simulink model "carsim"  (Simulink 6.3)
settings: Solver=ode3  StartTime=0.0  StopTime=130  RelTol=1e-3
libraries: simulink x2

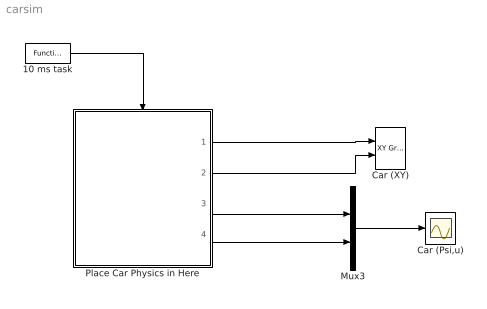
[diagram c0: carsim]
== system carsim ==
  10 ms task : simulink/Ports & Subsystems/Function-Call Generator  sample_time=0.01  numberOfIterations=1
  Car (Psi,u) : Scope
  Car (XY) : simulink/Sinks/XY Graph  xmin=-250  xmax=250  ymin=-250  ymax=250  st=-1
  Mux3 : Mux  Inputs=2
  Place Car Physics in Here : Subsystem  TreatAsAtomicUnit=on
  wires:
  10 ms task/1 -> Place Car Physics in Here/Trigger
  Place Car Physics in Here/3(psi) -> Mux3/1
  Place Car Physics in Here/1(x) -> Car (XY)/1
  Place Car Physics in Here/2(y) -> Car (XY)/2
  Place Car Physics in Here/4(u) -> Mux3/2
  Mux3/1 -> Car (Psi,u)/1

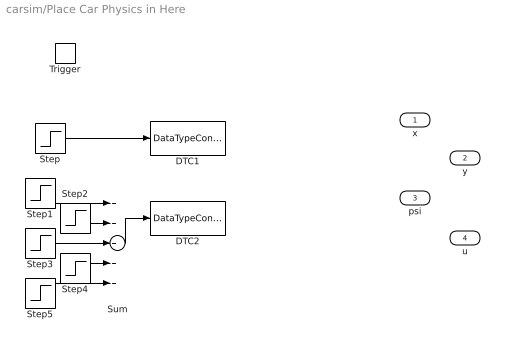
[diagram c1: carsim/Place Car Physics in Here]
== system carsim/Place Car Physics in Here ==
  Trigger : TriggerPort  TriggerType=function-call
  DTC1 : DataTypeConversion  OutDataTypeMode=single
  DTC2 : DataTypeConversion  OutDataTypeMode=single
  Step : Step  After=1000
  Step1 : Step  Time=30  After=2*pi/180
  Step2 : Step  Time=50  After=-4*pi/180
  Step3 : Step  Time=70  After=5*pi/180
  Step4 : Step  Time=83  After=-3*pi/180
  Step5 : Step  Time=110  After=0.7*pi/180
  Sum : Sum  Inputs=+++++
  x : Outport
  y : Outport  Port=2
  psi : Outport  Port=3
  u : Outport  Port=4
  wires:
  Step/1 -> DTC1/1
  Sum/1 -> DTC2/1
  DTC1/1 -> ?  "Fd"
  DTC2/1 -> ?  "delta"
  ? -> x/1  "x"
  ? -> y/1  "y"
  ? -> psi/1  "psi"
  ? -> u/1  "u"
  Step1/1 -> Sum/1
  Step2/1 -> Sum/2
  Step3/1 -> Sum/3
  Step4/1 -> Sum/4
  Step5/1 -> Sum/5
